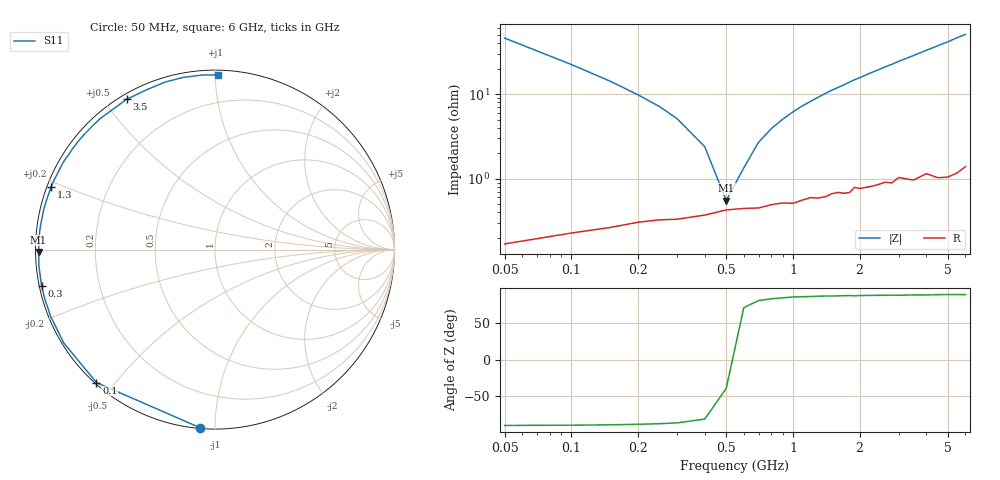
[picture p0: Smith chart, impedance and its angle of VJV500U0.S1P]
! Infineon Technologies  Discrete & RF Semiconductors
! BB 914
! Si Tuning Diode in SOT23
! VR = 0.5 V
! S-Parameters:  July  1999
# GHz  S  MA  R  50
!  f  S11
! GHz  MAG  ANG
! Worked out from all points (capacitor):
!   34 points, 50 MHz to 6 GHz, reference 50 ohm
!   read as one part to ground: C = 68.5 pF near 50 MHz
!   lowest |Z| = 551 mohm at 500 MHz (marker M1)
!   series resonance near 521.6 MHz, so ESL is about 1.4 nH
!   S11 on the Smith chart (normalised r, x): 50 MHz: 0.00, -0.92; 100 MHz: 0.00, -0.45; 300 MHz: 0.01, -0.10; 1.3 GHz: 0.01, +0.18; 3.5 GHz: 0.02, +0.57; 6 GHz: 0.03, +1.02
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0.05  0.9963 -94.7
0.1  0.9925 -131.7
0.15  0.9902 -148.3
0.2  0.9883 -157.8
0.25  0.9873 -163.8
0.3  0.987 -168.3
0.4  0.9853 -174.6
0.5  0.9831 -179.2
0.6  0.9824 177.1
0.7  0.9822 173.9
0.8  0.9806 171.1
1.1  0.9784 163.6
1.3  0.9774 159.2
1.5  0.975 154.9
1.6  0.9743 153.0
1.7  0.9752 151.1
1.9  0.9714 147.0
2.2  0.9719 141.5
2.4  0.971 138.1
2.6  0.9696 134.5
2.8  0.9708 131.4
3  0.9672 128.0
3.5  0.9714 120.4
4  0.9686 113.1
4.5  0.974 106.5
5  0.9757 100.5
5.5  0.9752 94.2
6  0.9731 89.1
